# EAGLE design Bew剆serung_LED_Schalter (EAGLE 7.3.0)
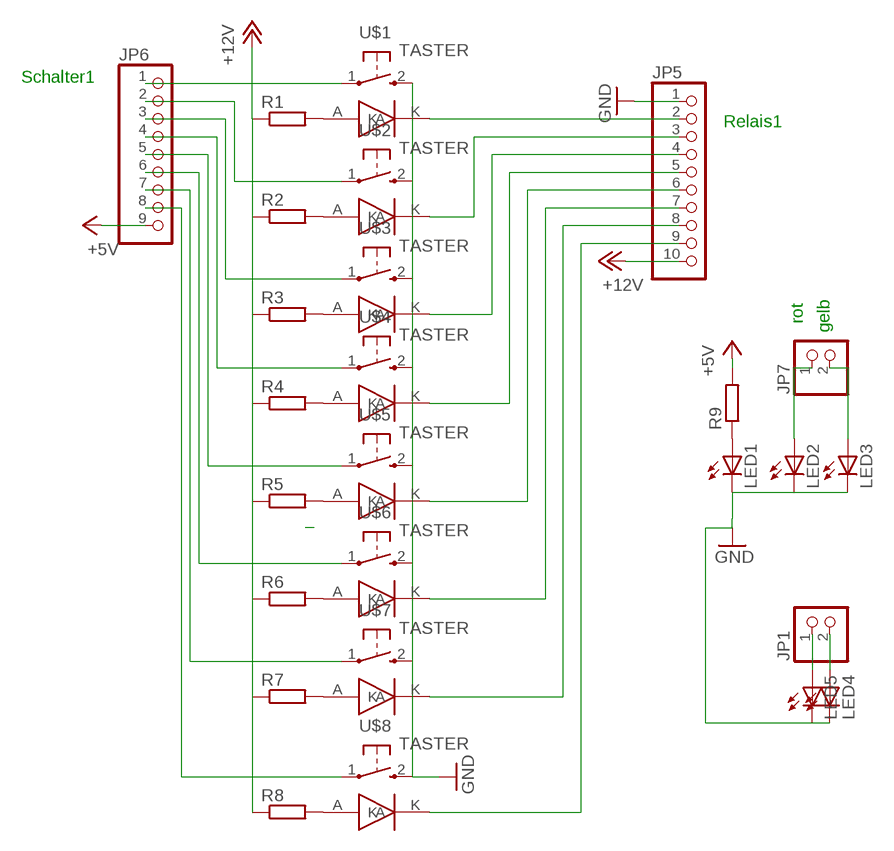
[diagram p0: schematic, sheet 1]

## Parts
JP1  PINHD-1X2  [1X02]
JP5  PINHD-1X10  [1X10]
JP6  PINHD-1X9  [1X09]
JP7  PINHD-1X2  [1X02]
LED1  LED3MM  [LED3MM]
LED2  LED3MM  [LED3MM]
LED3  LED3MM  [LED3MM]
LED4  LED3MM  [LED3MM]
LED5  LED3MM  [LED3MM]
R1  R-EU_R1206  [R1206]
R2  R-EU_R0603  [R0603]
R3  R-EU_R0603  [R0603]
R4  R-EU_R0603  [R0603]
R5  R-EU_R0603  [R0603]
R6  R-EU_R0603  [R0603]
R7  R-EU_R0603  [R0603]
R8  R-EU_R0603  [R0603]
R9  R-EU_R0603  [R0603]
U$1  TASTER  [TASTER]
U$2  TASTER  [TASTER]
U$3  TASTER  [TASTER]
U$4  TASTER  [TASTER]
U$5  TASTER  [TASTER]
U$6  TASTER  [TASTER]
U$7  TASTER  [TASTER]
U$8  TASTER  [TASTER]

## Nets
+5V: JP6.9 R9.2
+12V: JP5.10 R1.1 R2.1 R3.1 R4.1 R5.1 R6.1 R7.1 R8.1
GND: JP5.1 LED1.K(C) LED2.K(C) LED3.K(C) LED4.K(C) LED5.K(C) U$1.2(S) U$2.2(S) U$3.2(S) U$4.2(S) U$5.2(S) U$6.2(S) U$7.2(S) U$8.2(S)
N$1: JP6.1 U$1.1(P)
N$2: JP6.2 U$2.1(P)
N$3: JP6.3 U$3.1(P)
N$4: JP6.4 U$4.1(P)
N$5: JP6.5 U$5.1(P)
N$6: JP6.6 U$6.1(P)
N$7: JP6.7 U$7.1(P)
N$8: JP6.8 U$8.1(P)
N$9: JP5.2 U$1.K
N$10: JP5.3 U$2.K
N$11: JP5.4 U$3.K
N$12: JP5.5 U$4.K
N$13: JP5.6 U$5.K
N$14: JP5.7 U$6.K
N$15: JP5.8 U$7.K
N$16: JP5.9 U$8.K
N$17: R1.2 U$1.A
N$18: R2.2 U$2.A
N$19: R3.2 U$3.A
N$20: R4.2 U$4.A
N$21: R5.2 U$5.A
N$22: R6.2 U$6.A
N$23: R7.2 U$7.A
N$24: R8.2 U$8.A
N$26: JP1.1 LED5.A
N$27: LED1.A R9.1
N$28: JP7.1 LED2.A
N$29: JP7.2 LED3.A
N$30: JP1.2 LED4.A

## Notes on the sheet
- Schalter1
- Relais1
- rot
- gelb

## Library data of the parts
JP1 JP7 = pinhead:PINHD-1X2: PIN HEADER
JP5 = pinhead:PINHD-1X10: PIN HEADER
JP6 = pinhead:PINHD-1X9: PIN HEADER
LED1-LED5 = led:LED: LED
R1-R9 = rcl:R-EU_: RESISTOR, European symbol
U$1-U$8 = Ergaenzung:TASTER

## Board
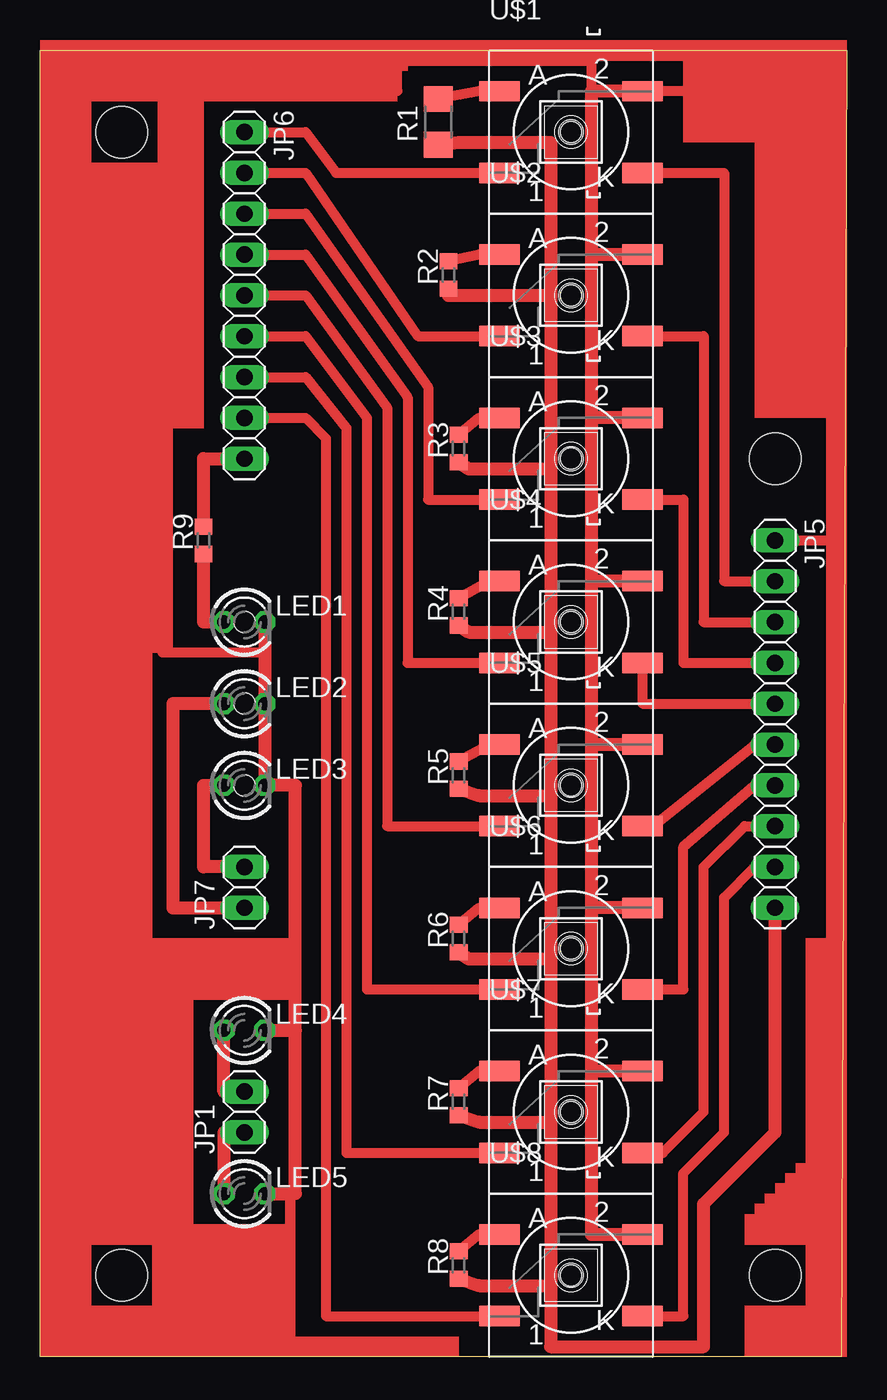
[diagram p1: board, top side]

Size 50.16 x 81.28 mm. Coordinates in mm from the lower left corner, seen from the top.
Outline: 0,81.28 50.16,81.28 49.85,0 0,0 0,81.28
Copper layers (1*16): Top 0.035mm / dielectric 1.5mm / Bottom 0.035mm
Design rules "default": minimum track width 10mil, minimum drill 24mil, track to track 8mil, track to pad 8mil, pad to pad 8mil, via to via 8mil, smd to smd 8mil, copper to edge 40mil, drill to drill 8mil, minimum pad ring 10mil, minimum via ring 8mil, stop-mask expansion 4mil, vias tented up to drill 0mil, thermal gap 10mil
Holes 3.2 mm at 5.08,76.2 5.08,5.08 45.72,55.88 45.72,5.08
Holes 1.3 mm at 33.02,76.2 33.02,66.04 33.02,55.88 33.02,45.72 33.02,35.56 33.02,25.4 33.02,15.24 33.02,5.08 12.7,35.56 12.7,40.64 12.7,45.72

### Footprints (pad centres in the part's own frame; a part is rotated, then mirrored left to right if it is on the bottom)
1X02 = drill 1.016 long: 1 -1.27,0; 2 1.27,0
1X10 = drill 1.016 long: 1 -11.43,0; 2 -8.89,0; 3 -6.35,0; 4 -3.81,0; 5 -1.27,0; 6 1.27,0; 7 3.81,0; 8 6.35,0; 9 8.89,0; 10 11.43,0
1X09 = drill 1.016 long: 1 -10.16,0; 2 -7.62,0; 3 -5.08,0; 4 -2.54,0; 5 0,0; 6 2.54,0; 7 5.08,0; 8 7.62,0; 9 10.16,0
LED3MM = drill 0.813 octagon: A -1.27,0; K 1.27,0
R1206 = smd 1.6 x 1.803: 1 -1.422,0; 2 1.422,0
R0603 = smd 1 x 1.1: 1 -0.85,0; 2 0.85,0
TASTER = smd 2.54 x 1.27: 1 -4.445,-2.54; 2 4.445,2.54; A -4.445,2.54; K 4.445,-2.54

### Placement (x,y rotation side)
JP1  12.7,15.24 90 top
JP5  45.72,39.37 270 top
JP6  12.7,66.04 270 top
JP7  12.7,29.21 90 top
LED1  12.7,45.72 0 top
LED2  12.7,40.64 0 top
LED3  12.7,35.56 0 top
LED4  12.7,20.32 0 top
LED5  12.7,10.16 0 top
R1  24.77,76.83 90 top
R2  25.4,67.31 90 top
R3  26.04,56.52 90 top
R4  26.04,46.35 90 top
R5  26.04,36.2 90 top
R6  26.04,26.04 90 top
R7  26.04,15.88 90 top
R8  26.04,5.71 90 top
R9  10.16,50.8 90 top
U$1  33.02,76.2 0 top
U$2  33.02,66.04 0 top
U$3  33.02,55.88 0 top
U$4  33.02,45.72 0 top
U$5  33.02,35.56 0 top
U$6  33.02,25.4 0 top
U$7  33.02,15.24 0 top
U$8  33.02,5.08 0 top

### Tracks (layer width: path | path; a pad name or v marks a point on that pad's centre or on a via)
+5V
  Top 0.813: R9.2 10.16,55.88 JP6.9
+12V
  Top 0.813: R1.1 26.04,75.56 31.75,75.56 31.75,66.04 | 31.75,66.04 31.75,55.24 | 31.75,55.24 31.75,45.09 | 31.75,45.09 31.75,34.92 | 31.75,34.92 31.75,24.77 | 31.75,24.77 31.75,14.61 | 31.75,14.61 31.75,4.45 | 31.75,4.45 31.75,0.64 41.27,0.64 41.27,9.53 45.72,13.97 JP5.10 | R2.1 25.4,66.04 31.75,66.04 | R3.1 26.67,55.24 31.75,55.24 | R4.1 26.67,45.09 31.75,45.09 | R5.1 27.3,34.92 31.75,34.92 | R6.1 26.67,24.77 31.75,24.77 | R7.1 27.3,14.61 31.75,14.61 | R8.1 27.3,4.45 31.75,4.45
GND
  Top 0.61: 13.97,43.81 7.62,43.81 7.62,78.74 22.23,78.74 22.23,80.64 34.29,80.64 34.29,78.74 | JP5.1 49.53,50.8 49.53,78.74 36.83,78.74
  Top 0.813: LED1.K 13.97,43.81 LED2.K LED3.K 15.88,35.56 15.88,20.32 | U$1.2 36.83,78.74 34.29,78.74 34.29,68.58 | 34.29,68.58 34.29,58.42 | 34.29,58.42 34.29,48.26 | 34.29,48.26 34.29,38.1 | 34.29,38.1 34.29,27.94 | 34.29,27.94 34.29,17.78 | 34.29,17.78 34.29,7.62 U$8.2 | U$7.2 34.29,17.78 | U$6.2 34.29,27.94 | U$5.2 34.29,38.1 | U$4.2 34.29,48.26 | U$3.2 34.29,58.42 | U$2.2 34.29,68.58 | LED4.K 15.88,20.32 | LED5.K 15.88,10.16 15.88,20.32
N$1
  Top 0.61: JP6.1 16.51,76.2 18.41,73.66 U$1.1
N$2
  Top 0.61: JP6.2 16.51,73.66 23.5,63.5 U$2.1
N$3
  Top 0.61: U$3.1 24.13,53.34 24.13,60.33 16.51,71.12 JP6.3
N$4
  Top 0.61: U$4.1 22.86,43.18 22.86,59.69 16.51,68.58 JP6.4
N$5
  Top 0.61: JP6.5 16.51,66.04 21.59,59.05 21.59,33.02 U$5.1
N$6
  Top 0.61: U$6.1 20.32,22.86 20.32,58.42 16.51,63.5 JP6.6
N$7
  Top 0.61: JP6.7 16.51,60.96 19.05,57.78 19.05,12.7 U$7.1
N$8
  Top 0.61: JP6.8 16.51,58.42 17.78,57.15 17.78,2.54 U$8.1
N$9
  Top 0.61: U$1.K 42.55,73.66 42.55,48.26 JP5.2
N$10
  Top 0.61: U$2.K 41.27,63.5 41.27,45.72 JP5.3
N$11
  Top 0.61: U$3.K 40.01,53.34 40.01,43.18 JP5.4
N$12
  Top 0.61: U$4.K 37.47,40.64 JP5.5
N$13
  Top 0.61: U$5.K 38.1,33.02 44.45,38.1 JP5.6
N$14
  Top 0.61: U$6.K 40.01,22.86 40.01,31.75 44.45,35.56 JP5.7
N$15
  Top 0.61: JP5.8 43.81,33.02 41.27,30.48 41.27,15.24 38.73,12.7 U$7.K
N$16
  Top 0.61: U$8.K 40.01,2.54 40.01,11.43 42.55,13.97 42.55,28.57 44.45,30.48 JP5.9
N$17
  Top 0.61: U$1.A 27.3,78.74 R1.2
N$18
  Top 0.61: U$2.A 27.3,68.58 R2.2
N$19
  Top 0.61: U$3.A 27.3,58.42 R3.2
N$20
  Top 0.61: U$4.A 27.94,48.26 R4.2
N$21
  Top 0.61: U$5.A 27.94,38.1 R5.2
N$22
  Top 0.61: U$6.A 27.3,27.94 R6.2
N$23
  Top 0.61: U$7.A 27.3,17.78 R7.2
N$24
  Top 0.61: U$8.A 27.3,7.62 R8.2
N$26
  Top 0.813: JP1.1 11.43,13.97 LED5.A
N$27
  Top 0.813: LED1.A 10.16,45.72 R9.1
N$28
  Top 0.813: LED2.A 8.26,40.64 8.26,27.94 JP7.1
N$29
  Top 0.813: JP7.2 10.16,30.48 10.16,35.56 LED3.A
N$30
  Top 0.813: JP1.2 11.43,16.51 LED4.A
(copper drawn outside any net)
  shapes: Top area x38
